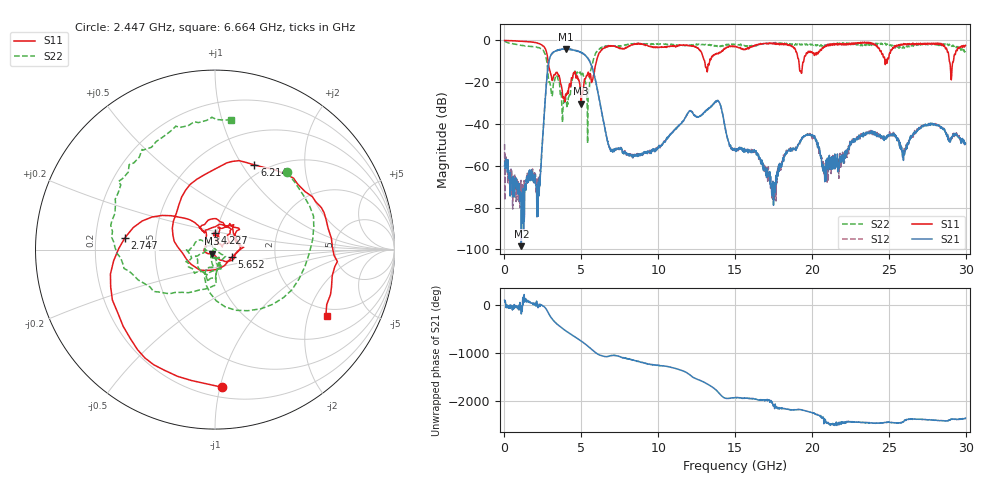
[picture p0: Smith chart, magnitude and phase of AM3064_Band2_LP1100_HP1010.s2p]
# Hz S DB R 50.0
!freq dBS11 angS11 dBS21 angS21 dBS12 angS12 dBS22 angS22
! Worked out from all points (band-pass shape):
!   1600 points, 10 MHz to 29.98 GHz, reference 50 ohm
!   highest |S21| = -4.08 dB at 4.002 GHz (marker M1); lowest = -98.4 dB at 1.097 GHz (marker M2)
!   |S21| within 3 dB of the highest: 3.021 GHz to 5.236 GHz (2.216 GHz wide, 53.7 % of centre)
!   lowest |S11| = -30.4 dB at 4.996 GHz (marker M3), VSWR 1.06, Z = 48.1 - j2.26 ohm
!   |S11| at or under -10 dB: 2.837 GHz to 5.985 GHz (3.149 GHz wide, 71.4 % of centre); 13.02 GHz to 13.34 GHz (321.2 MHz wide, 2.44 % of centre); 19.15 GHz to 19.47 GHz (315.5 MHz wide, 1.63 % of centre)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
!   |S22| runs from -49.2 to -0.3 dB; largest |S21 - S12| = 0.015
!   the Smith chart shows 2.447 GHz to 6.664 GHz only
!   S11 on the Smith chart (normalised r, x): 2.447 GHz: 0.27, -1.01; 2.747 GHz: 0.33, +0.06; 4.227 GHz: 0.98, +0.18; 5.652 GHz: 1.20, -0.10; 6.214 GHz: 0.88, +1.13; 6.664 GHz: 1.70, -2.66
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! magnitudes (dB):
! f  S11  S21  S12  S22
! 10 MHz  0.0  -59.9  -49.6  -0.3
! 1.097 GHz  -0.4  -98.4  -74.5  -2.4
! 2.184 GHz  -1.4  -84.2  -68.3  -3.5
! 2.447 GHz  -2.3  -50.8  -50.5  -4.6
! 2.747 GHz  -5.9  -19.0  -19.0  -9.8
! 4.002 GHz  -25.6  -4.1  -4.1  -29.0
! 4.227 GHz  -20.8  -4.3  -4.2  -26.2
! 4.996 GHz  -30.4  -5.8  -5.8  -17.2
! 5.015 GHz  -27.1  -6.0  -5.9  -17.1
! 5.389 GHz  -16.6  -8.3  -8.3  -32.9
! 5.652 GHz  -19.8  -11.8  -11.8  -13.3
! 6.214 GHz  -5.7  -30.1  -30.0  -3.9
! 6.664 GHz  -2.8  -46.8  -46.6  -2.7
! 10 GHz  -3.4  -51.3  -51.4  -1.8
! 13.82 GHz  -6.1  -28.8  -28.9  -2.5
! 15 GHz  -2.8  -52.7  -52.4  -1.9
! 17.52 GHz  -1.6  -74.8  -77.0  -1.2
! 18.3 GHz  -1.6  -53.7  -53.9  -1.9
! 19.99 GHz  -5.4  -45.1  -45.8  -1.8
! 20.82 GHz  -3.0  -62.6  -61.0  -2.3
! 25 GHz  -8.3  -45.1  -45.7  -1.8
! 29.98 GHz  -2.4  -49.3  -49.1  -4.7
